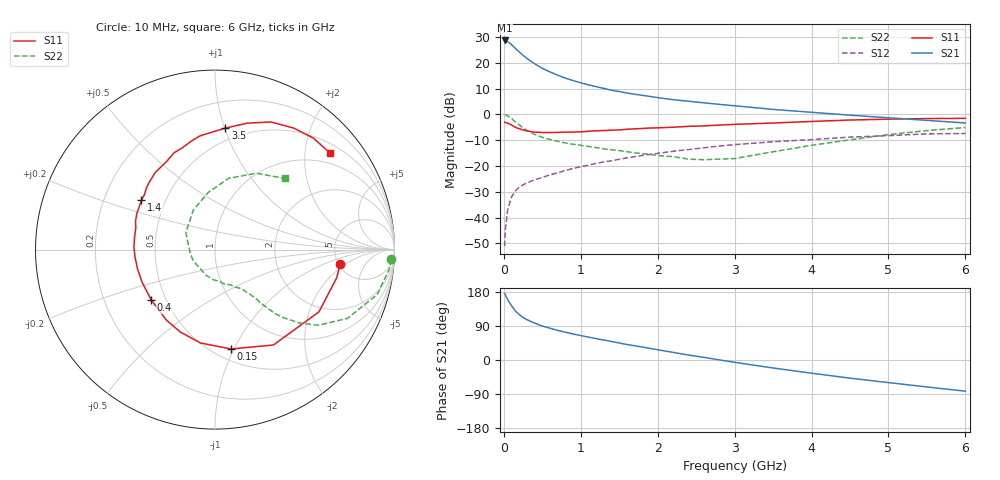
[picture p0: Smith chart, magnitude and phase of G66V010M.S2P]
! SIEMENS Small Signal Semiconductors
! BFG193
! Si NPN RF Bipolar Junction Transistor in SOT223
! VCE = 6 V  IC = 10 mA
! Common Emitter S-Parameters:  August  1996
# GHz  S  MA  R  50
!  f  S11  S21  S12  S22
! GHz  MAG  ANG  MAG  ANG  MAG  ANG  MAG  ANG
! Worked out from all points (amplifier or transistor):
!   36 points, 10 MHz to 6 GHz, reference 50 ohm
!   highest |S21| = 28.6 dB at 10 MHz (marker M1)
!   |S21| within 3 dB of that: start of sweep to 147.7 MHz
!   unconditionally stable (mu >= 1): 905 MHz to 2.551 GHz
!   at 250 MHz: K = 0.53, MSG = 25.1 dB, |S12| = -27.3 dB
!   at 1.4 GHz: K = 1.07, MAG = 12.1 dB, |S12| = -18.0 dB
!   at 6 GHz: K = 0.86, MSG = 2.0 dB, |S12| = -7.4 dB
!   S11 on the Smith chart (normalised r, x): 10 MHz: 5.20, -1.63; 150 MHz: 0.60, -0.98; 400 MHz: 0.42, -0.29; 1.4 GHz: 0.37, +0.27; 3.5 GHz: 0.40, +1.01; 6 GHz: 0.71, +2.56
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0.01  0.7027 -6.5  26.96 175.3  0.0028 91.8  0.984 -3.2
0.02  0.6961 -13.0  26.7 172.0  0.0059 83.2  0.9772 -6.4
0.05  0.6751 -30.9  25.52 158.9  0.0142 76.6  0.9374 -15.5
0.1  0.6233 -58.5  22.48 143.2  0.0251 66.6  0.8324 -27.4
0.15  0.5608 -80.8  18.94 129.2  0.0331 57.8  0.7149 -36.1
0.2  0.5264 -98.9  16.23 120.1  0.0386 54.5  0.6247 -40.9
0.25  0.4981 -112.9  13.93 112.2  0.0432 51.9  0.5446 -44.5
0.3  0.4768 -124.7  12.12 106.3  0.047 51.5  0.4907 -46.8
0.4  0.4526 -141.7  9.543 97.4  0.0539 50.5  0.4093 -49.0
0.5  0.4452 -156.0  7.786 89.7  0.0601 50.2  0.3588 -50.1
0.6  0.445 -166.2  6.617 83.8  0.0674 51.3  0.3259 -51.4
0.7  0.4476 -174.7  5.734 78.2  0.074 51.2  0.3008 -53.1
0.9  0.4536 171.3  4.507 68.7  0.0895 50.9  0.2633 -55.7
1.1  0.4705 160.2  3.722 60.5  0.104 50.1  0.2385 -61.4
1.4  0.4934 146.1  2.934 48.9  0.1263 46.9  0.2061 -70.2
1.7  0.5231 134.9  2.451 37.6  0.1514 43.2  0.1795 -81.3
2.2  0.5623 118.2  1.925 20.1  0.1925 34.6  0.1517 -109.6
2.8  0.6196 102.1  1.561 0.3  0.2432 23.0  0.1357 -155.7
3.5  0.6796 85.1  1.246 -21.1  0.2943 7.1  0.1883 149.8
4.5  0.7765 66.3  0.964 -47.9  0.362 -12.6  0.321 96.7
5.5  0.8283 48.7  0.764 -71.1  0.4178 -37.1  0.4842 61.5
6  0.8366 40.2  0.681 -82.4  0.4264 -51.2  0.5556 45.5
